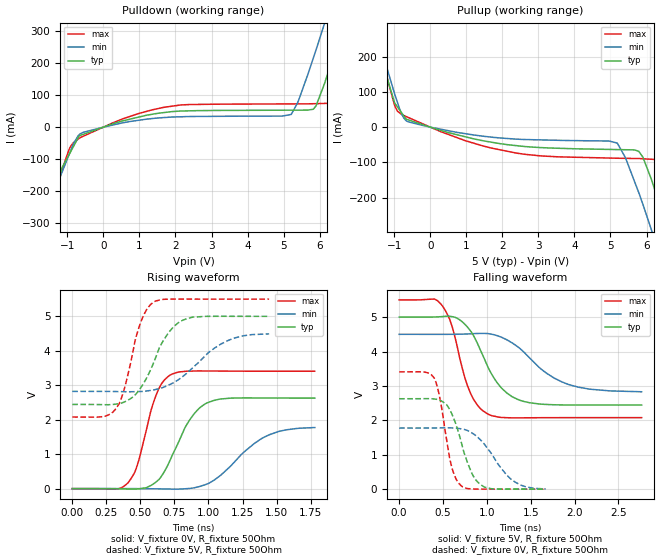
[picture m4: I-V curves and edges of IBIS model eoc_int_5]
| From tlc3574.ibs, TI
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|   eoc_int_5 Model
[Model]   eoc_int_5
Model_type   Output
Polarity   Non-Inverting
Vmeas = 2.5
Vref = 2.5
Cref = 10pF
Rref = 50
|   typ   min   max
C_comp   1.437e-12   1.431e-12   1.465e-12
[Voltage Range]   5   4.5   5.5
|Ambient Temperature   25   85   -40
|Junction Temperature
[Temperature Range]   27   125   -40
[Pullup Reference]   5   4.5   5.5
[Pulldown Reference]   0   0   0
[Power Clamp Reference]   5   4.5   5.5
[GND Clamp Reference]   0   0   0
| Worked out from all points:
|   slope of the pulldown table from 0 to 0.75 V, typ, clamps not added: 29.7 ohm
|   slope of the pullup table from 0 to 0.75 V, typ, clamps not added: 34.5 ohm
|   falling waveform, V_fixture 5V, R_fixture 50Ohm: 20-80 % time 320ps typ, 482ps min, 226ps max; typ from 5 V to 2.44 V
|   rising waveform, V_fixture 0V, R_fixture 50Ohm: 20-80 % time 201ps typ, 298ps min, 140ps max; typ from 0 V to 2.63 V
|   rising waveform, V_fixture 5V, R_fixture 50Ohm: 20-80 % time 193ps typ, 298ps min, 129ps max; typ from 2.44 V to 5 V
|   falling waveform, V_fixture 0V, R_fixture 50Ohm: 20-80 % time 203ps typ, 316ps min, 138ps max; typ from 2.63 V to 0.001 V
[Pulldown]
|   Voltage   I(typ)   I(min)   I(max)
-5V       -1.586A    -1.466A    -1.707A
-2.365V   -567.9mA   -532.7mA   -623.3mA
-1.375V   -203.6mA   -204.7mA   -220.3mA
-946mV    -84.33mA   -83.63mA   -67.92mA
-549mV    -21.97mA   -15.89mA   -27.71mA
1.672V    45.28mA    29.76mA    61.61mA
5.207V    52.86mA    39.44mA    72.37mA
5.825V    55.8mA     215.6mA    72.98mA
6.13V     134.2mA    321.1mA    73.87mA
6.835V    386.2mA    574.9mA    211.9mA
7.835V    769mA      948.9mA    600mA
10V       1.626A     1.782A     1.474A
[Pullup]
|   Voltage   I(typ)   I(min)   I(max)
-5V       1.654A     1.613A     1.708A
-2.61V    688.9mA    688.7mA    710.2mA
-1.375V   206.6mA    227.9mA    204.9mA
-984.5mV  67.92mA    92.58mA    60.54mA
-616.5mV  20.75mA    15.24mA    27.69mA
2.376V    -52.32mA   -33.96mA   -73.36mA
5.184V    -63.61mA   -45.16mA   -88.18mA
5.785V    -68.59mA   -185.9mA   -89.02mA
6.13V     -146.7mA   -289.6mA   -91.02mA
6.6V      -298.9mA   -440.8mA   -158.6mA
6.891V    -401.1mA   -537mA     -261.1mA
10V       -1.602A    -1.646A    -1.538A
[Ramp]
R_load = 50
|   typ   min   max
dV/dt_r   1.5762/2.00599e-10   1.06552/2.97455e-10   2.0451/1.39468e-10
dV/dt_f   1.53356/3.19509e-10   1.00623/4.82019e-10   2.05295/2.25803e-10
[Falling Waveform]
V_fixture = 5V
V_fixture_min = 4.5V
V_fixture_max = 5.5V
R_fixture = 50Ohm
|   Time   V(typ)   V(min)   V(max)
0s        5V         4.5V       5.5V
400ps     5.003V     4.5V       5.525V
485ps     5.015V     4.499V     5.354V
595ps     5.017V     4.5V       4.797V
810ps     4.612V     4.514V     2.811V
1.025ns   3.482V     4.516V     2.167V
1.225ns   2.801V     4.345V     2.078V
1.425ns   2.547V     3.977V     2.073V
1.94ns    2.446V     3.036V     2.078V
2.765ns   2.444V     2.83V      2.079V
[Rising Waveform]
V_fixture = 0V
V_fixture_min = 0V
V_fixture_max = 0V
R_fixture = 50Ohm
|   Time   V(typ)   V(min)   V(max)
0s        243pV      590pV      222.7pV
345ps     -4.235mV   513.8uV    570.6uV
410ps     -10.7mV    588uV      176.1mV
480ps     -7.506mV   -543.2uV   714.8mV
620ps     209.9mV    -5.836mV   2.759V
730ps     933.5mV    -13.24mV   3.32V
860ps     1.982V     5.396mV    3.411V
1ns       2.505V     150.9mV    3.414V
1.41ns    2.631V     1.496V     3.408V
1.78ns    2.627V     1.773V     3.408V
[Rising Waveform]
V_fixture = 5V
V_fixture_min = 4.5V
V_fixture_max = 5.5V
R_fixture = 50Ohm
|   Time   V(typ)   V(min)   V(max)
0s        2.444V     2.823V     2.078V
230ps     2.437V     2.822V     2.091V
325ps     2.455V     2.818V     2.348V
385ps     2.52V      2.813V     2.937V
495ps     2.884V     2.818V     4.744V
595ps     3.632V     2.864V     5.409V
700ps     4.487V     2.991V     5.498V
815ps     4.894V     3.266V     5.501V
1.145ns   5.001V     4.302V     5.5V
1.445ns   5V         4.491V     5.5V
[Falling Waveform]
V_fixture = 0V
V_fixture_min = 0V
V_fixture_max = 0V
R_fixture = 50Ohm
|   Time   V(typ)   V(min)   V(max)
0s        2.627V     1.776V     3.409V
295ps     2.63V      1.776V     3.401V
400ps     2.62V      1.779V     3.231V
465ps     2.585V     1.781V     2.637V
595ps     2.219V     1.78V      691.2mV
710ps     1.348V     1.751V     93.29mV
835ps     430.4mV    1.626V     5.786mV
965ps     72.27mV    1.327V     602.3uV
1.275ns   2.585mV    292.4mV    -67.42uV
1.67ns    542.1uV    6.453mV    209.3uV
